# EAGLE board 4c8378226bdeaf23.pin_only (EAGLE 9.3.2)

Size 102.87 x 46.99 mm. Coordinates in mm from the lower left corner, seen from the top.
Outline: 100.33,46.99 arc-90 102.87,44.45
Outline: 102.87,44.45 102.87,2.54 arc-90 100.33,0 2.54,0 arc-90 0,2.54 0,44.45 arc-90 2.54,46.99 100.33,46.99
Outline: 102.87,44.45 arc90 100.33,46.99
Copper layers (1*16): Top 0.035mm / dielectric 1.5mm / Bottom 0.035mm
Design rules "adafruit": minimum track width 8mil, minimum drill 15.5mil, track to track 8mil, track to pad 8mil, pad to pad 8mil, via to via 8mil, smd to smd 8mil, copper to edge 10mil, drill to drill 8mil, minimum pad ring 10mil, minimum via ring 8mil, stop-mask expansion 2mil, vias tented up to drill 20mil, thermal gap 10mil

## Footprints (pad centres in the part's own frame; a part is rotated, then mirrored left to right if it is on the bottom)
1X12_ROUND_76MIL = drill 1 pad 1.93: 1 -13.97,0; 2 -11.43,0; 3 -8.89,0; 4 -6.35,0; 5 -3.81,0; 6 -1.27,0; 7 1.27,0; 8 3.81,0; 9 6.35,0; 10 8.89,0; 11 11.43,0; 12 13.97,0
1X16_ROUND_76MIL = drill 1 pad 1.93: 1 -19.05,0; 2 -16.51,0; 3 -13.97,0; 4 -11.43,0; 5 -8.89,0; 6 -6.35,0; 7 -3.81,0; 8 -1.27,0; 9 1.27,0; 10 3.81,0; 11 6.35,0; 12 8.89,0; 13 11.43,0; 14 13.97,0; 15 16.51,0; 16 19.05,0
FEATHERWING_DIM = drill 1 pad 1.778: 1 6.35,1.27; 2 8.89,1.27; 3 11.43,1.27; 4 13.97,1.27; 5 16.51,1.27; 6 19.05,1.27; 7 21.59,1.27; 8 24.13,1.27; 9 26.67,1.27; 10 29.21,1.27; 11 31.75,1.27; 12 34.29,1.27; 13 36.83,1.27; 14 39.37,1.27; 15 41.91,1.27; 16 44.45,1.27; 17 44.45,21.59; 18 41.91,21.59; 19 39.37,21.59; 20 36.83,21.59; 21 34.29,21.59; 22 31.75,21.59; 23 29.21,21.59; 24 26.67,21.59; 25 24.13,21.59; 26 21.59,21.59; 27 19.05,21.59; 28 16.51,21.59 | drill 2.5 pad 3.81: P$1 2.54,20.32; P$2 2.54,2.54 | hole 2.54: 48.26,20.32; 48.26,2.54

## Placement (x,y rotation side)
JP1  [1X12_ROUND_76MIL]  30.48,19.05 0 top
JP2  [1X16_ROUND_76MIL]  25.4,27.94 180 top
JP3  [1X16_ROUND_76MIL]  25.4,3.81 180 top
JP4  [1X12_ROUND_76MIL]  30.48,43.18 0 top
JP5  [1X12_ROUND_76MIL]  82.55,19.05 0 top
JP6  [1X16_ROUND_76MIL]  77.47,3.81 180 top
JP7  [1X12_ROUND_76MIL]  82.55,43.18 0 top
JP8  [1X16_ROUND_76MIL]  77.47,27.94 180 top
MS1  FEATHERWING_NODIM  [FEATHERWING_DIM]  0,0 0 top
MS2  FEATHERWING_NODIM  [FEATHERWING_DIM]  0,24.13 0 top
MS3  FEATHERWING_NODIM  [FEATHERWING_DIM]  52.07,0 0 top
MS4  FEATHERWING_NODIM  [FEATHERWING_DIM]  52.07,24.13 0 top
U$2  [FEATHERLOGO_MED]  67.31,33.21 0 top

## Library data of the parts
JP1-JP8 MS1-MS4 = microbuilder
U$2 = silks

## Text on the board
tPlace: bat | en | usb | scl | sda | bat | en | usb | scl | sda | Quad 2x2 / FeatherWing | rst | 3vo | gnd | sck | mosi | miso | rx | tx | rst | 3vo | gnd | sck | mosi | miso | rx | tx | bat | en | usb | scl | sda | bat | en | usb | scl | sda | rst | 3vo | gnd | sck | mo | mi | rx | tx | rst | 3vo | gnd | sck | mo | mi | rx | tx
